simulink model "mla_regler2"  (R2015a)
settings: Solver=ode5  StartTime=0.0  StopTime=10  FixedStep=0.0001  RelTol=1e-3
PreLoadFcn:
  | MLA_Sensor1 = load('mla_sensor1.dat');
libraries: libmla x1, simulink_need_slupdate x1, slrtlib x1

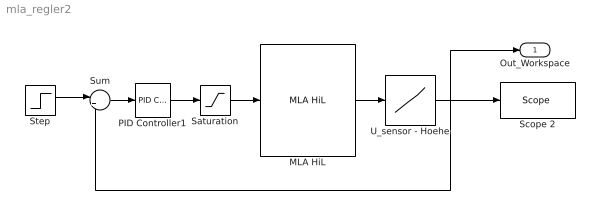
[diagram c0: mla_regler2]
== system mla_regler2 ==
  MLA HiL : libmla/MLA HiL  SystemSampleTime=-1
  PID Controller1 : simulink_need_slupdate/PID Controller  P=9000  I=2000  D=100
  Saturation : Saturate  UpperLimit=3  LowerLimit=-3
  Scope 2 : slrtlib/Displays and Logging/Scope   scopeno=1  scopetype=Target  autostart=on  viewmode=Graphical sliding  formatstr='%15.6f'  grid=on  ylimits=[0 0.132]  nosamples=1000  noprepostsamples=0  interleave=100  triggermode=FreeRun  triggersignal=1  trigsignalfromport=off  triggerlevel=0.0  triggerslope=Either  triggerscope=1  triggersample=0  filename=data.dat  mode=Lazy  writesize=512  autorestart=off  dynamicfilemode=off  maxwritefilesize=512*1024^2
  Step : Step  Time=0.1  After=0.02  SampleTime=0
  Sum : Sum  Inputs=|+-
  U_sensor - Hoehe : Lookup  InputValues=MLA_Sensor1(:,1)  Table=MLA_Sensor1(:,2)
  Out_Workspace : Outport
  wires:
  U_sensor - Hoehe/1 -> Scope 2/1, Sum/2, Out_Workspace/1
  Saturation/1 -> MLA HiL/1
  MLA HiL/1 -> U_sensor - Hoehe/1
  PID Controller1/1 -> Saturation/1
  Sum/1 -> PID Controller1/1
  Step/1 -> Sum/1
